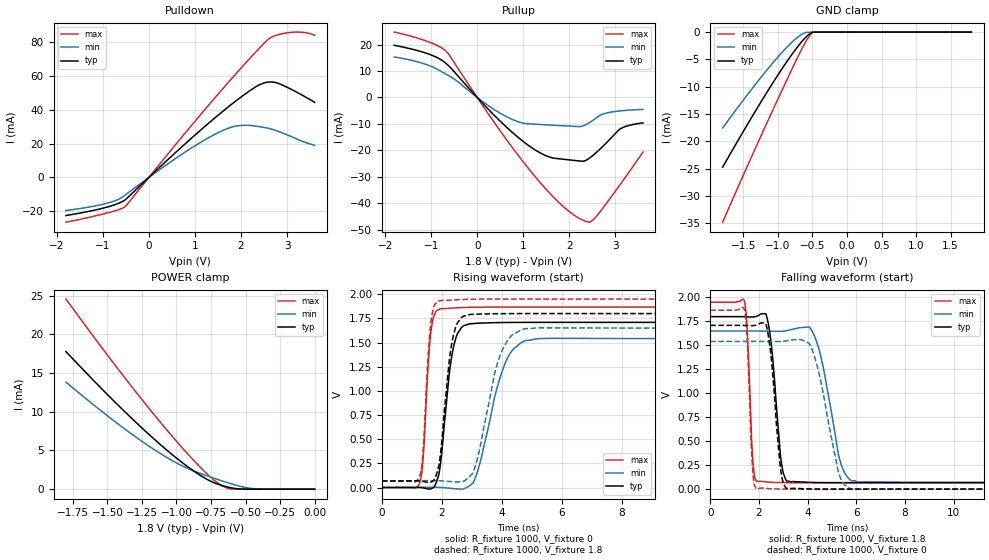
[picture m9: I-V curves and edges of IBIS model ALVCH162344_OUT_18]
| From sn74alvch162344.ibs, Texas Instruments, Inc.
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[Model]   ALVCH162344_OUT_18
Model_type  3-state
Enable   Active-Low
Vref =   0
Rref =   1000
Cref =   30p
Vmeas =   0.9
| variable   typ   min   max
C_comp   3.79pF   3.08pF   4.13pF
| C_pullup   2.49pF   1.20pF   4.61pF
| C_pulldown   1.14pF   0.73pF   1.99pF
| C_tri-state   3.79pF   3.08pF   4.13pF
[Temperature Range]   40   100   -40
| Ambient temperature   25   85   -40
[Voltage range]   1.8   1.65   1.95
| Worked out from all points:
|   slope of the pulldown table from 0 to 0.27 V, typ, clamps not added: 39.1 ohm
|   slope of the pullup table from 0 to 0.27 V, typ, clamps not added: 54.3 ohm
|   GND clamp passes 1 mA (typ) near -0.60 V on its own axis
|   POWER clamp passes 1 mA (typ) near -0.75 V on its own axis
|   rising waveform, R_fixture 1000, V_fixture 0: 20-80 % time 347ps typ, 732ps min, 205ps max; typ from 0 V to 1.71 V
|   falling waveform, R_fixture 1000, V_fixture 1.8: 20-80 % time 331ps typ, 662ps min, 179ps max; typ from 1.8 V to 0.067 V
|   rising waveform, R_fixture 1000, V_fixture 1.8: 20-80 % time 333ps typ, 654ps min, 202ps max; typ from 0.067 V to 1.8 V
|   falling waveform, R_fixture 1000, V_fixture 0: 20-80 % time 331ps typ, 716ps min, 170ps max; typ from 1.71 V to 0 V
[GND Clamp]
| ALVCH162344_OUT_18
|   Voltage   I(typ)   I(min)   I(max)
-1.8V     -24.75mA   -17.57mA   -34.84mA
-1.285V   -13.63mA   -8.929mA   -20.14mA
-1.08V    -9.446mA   -5.745mA   -14.47mA
-905mV    -6.056mA   -3.242mA   -9.706mA
-770mV    -3.623mA   -1.546mA   -6.073mA
-660mV    -1.839mA   -456.9uA   -3.236mA
-565mV    -568.6uA   -30.9uA    -1.109mA
-500mV    -40.16uA   -16.84uA   -114.6uA
-420mV    -2.964uA   -7.709uA   -1.366uA
1.8V      58.66pA    10.7nA     26.21pA
[POWER Clamp]
| ALVCH162344_OUT_18
|   Voltage   I(typ)   I(min)   I(max)
-1.8V     17.77mA    13.82mA    24.55mA
-1.44V    11.16mA    8.654mA    15.91mA
-1.15V    6.28mA     4.979mA    9.36mA
-1.015V   4.229mA    3.53mA     6.494mA
-900mV    2.655mA    2.525mA    4.186mA
-800mV    1.484mA    1.86mA     2.332mA
-715mV    735uA      1.33mA     985.6uA
-655mV    395.4uA    974.2uA    302.6uA
-605mV    178.9uA    695.8uA    24.81uA
-505mV    10.18uA    234.3uA    453nA
-425mV    558.3nA    44.67uA    18.74nA
-16.28fV  58.66pA    258.3pA    31.66pA
[Pulldown]
| ALVCH162344_OUT_18
|   Voltage   I(typ)   I(min)   I(max)
-1.8V     -22.48mA   -19.52mA   -26.42mA
-905mV    -17.49mA   -15.19mA   -20.95mA
-660mV    -15.29mA   -12.91mA   -19.09mA
-500mV    -12.91mA   -10.07mA   -16.79mA
660mV     16.68mA    12.65mA    22mA
1.47V     35.99mA    25.98mA    48.15mA
1.91V     45.59mA    30.44mA    61.8mA
2.415V    54.88mA    29.9mA     76.77mA
2.625V    56.36mA    28.8mA     82.2mA
2.885V    54.7mA     26.44mA    84.8mA
3.275V    49.39mA    21.93mA    85.78mA
3.6V      44.35mA    18.98mA    83.95mA
[Pullup]
| ALVCH162344_OUT_18
|   Voltage   I(typ)   I(min)   I(max)
-1.8V     19.73mA    15.31mA    24.72mA
-1.055V   16.43mA    12.16mA    21.02mA
-665mV    12.68mA    8.713mA    17.29mA
465mV     -8.372mA   -5.6mA     -11.78mA
1.115V    -18.15mA   -9.96mA    -26.89mA
1.59V     -22.62mA   -10.43mA   -36.47mA
2.27V     -24.1mA    -10.91mA   -46.19mA
2.44V     -22.89mA   -9.483mA   -47.15mA
2.565V    -21.14mA   -8.016mA   -45.39mA
2.755V    -18.03mA   -6.129mA   -41.21mA
3.105V    -11.9mA    -5.072mA   -32.9mA
3.6V      -9.595mA   -4.534mA   -20.62mA
[Ramp]
| ALVCH162344_OUT_18
| variable   typ   min   max
dV/dt_r   1.04/3.78E-10   0.94/7.80E-10   1.13/2.09E-10
dV/dt_f   1.06/3.45E-10   0.97/7.06E-10   1.15/1.95E-10
R_load = 1000
[Rising Waveform]
| ALVCH162344_OUT_18
R_fixture =   1000
C_fixture =   0
L_fixture =   0
V_fixture =   0
V_fixture_min = 0
V_fixture_max = 0
|   Time   V(typ)   V(min)   V(max)
0s        23.14uV    37.1uV     16.41uV
1.265ns   1.49mV     443.1uV    50.96mV
1.38ns    -3.025mV   1.424mV    312.9mV
1.635ns   -13.16mV   2.091mV    1.605V
1.955ns   243.9mV    885.8uV    1.85V
2.375ns   1.429V     -10.55mV   1.857V
2.915ns   1.693V     15.15mV    1.865V
4.115ns   1.708V     1.288V     1.867V
4.83ns    1.709V     1.522V     1.867V
24.99ns   1.709V     1.541V     1.867V
[Falling Waveform]
| ALVCH162344_OUT_18
R_fixture =   1000
C_fixture =   0
L_fixture =   0
V_fixture =   1.8
V_fixture_min = 1.65
V_fixture_max = 1.95
|   Time   V(typ)   V(min)   V(max)
0s        1.8V       1.65V      1.95V
1.405ns   1.799V     1.65V      1.963V
1.745ns   1.796V     1.65V      332.3mV
1.915ns   1.804V     1.65V      78.89mV
2.395ns   1.716V     1.648V     73.8mV
2.895ns   336.1mV    1.646V     68.42mV
3.17ns    81.25mV    1.655V     67.67mV
4.28ns    69.18mV    1.601V     67.01mV
5.82ns    67.3mV     87.47mV    67.19mV
24.99ns   67.42mV    70.3mV     67.21mV
[Rising Waveform]
| ALVCH162344_OUT_18
R_fixture =   1000
C_fixture =   0
L_fixture =   0
V_fixture =   1.8
V_fixture_min = 1.65
V_fixture_max = 1.95
|   Time   V(typ)   V(min)   V(max)
0s        67.38mV    70.2mV     67.19mV
1.265ns   68.15mV    70.35mV    121.6mV
1.375ns   63.91mV    71.16mV    377.1mV
1.62ns    54.23mV    71.39mV    1.667V
1.885ns   205.2mV    70.09mV    1.932V
2.355ns   1.528V     60.34mV    1.941V
2.905ns   1.789V     105.3mV    1.948V
3.95ns    1.799V     1.37V      1.95V
4.755ns   1.8V       1.641V     1.95V
24.99ns   1.8V       1.65V      1.95V
[Falling Waveform]
| ALVCH162344_OUT_18
R_fixture =   1000
C_fixture =   0
L_fixture =   0
V_fixture =   0
V_fixture_min = 0
V_fixture_max = 0
|   Time   V(typ)   V(min)   V(max)
0s        1.709V     1.541V     1.867V
1.4ns     1.708V     1.541V     1.879V
1.735ns   1.706V     1.541V     238.5mV
1.905ns   1.713V     1.541V     579uV
2.365ns   1.638V     1.541V     6.197mV
2.88ns    228.7mV    1.541V     997.2uV
3.145ns   6.755mV    1.548V     356.6uV
4.16ns    1.561mV    1.472V     -205.1uV
5.765ns   -147.9uV   4.211mV    -18.49uV
24.99ns   237.8nV    402.4nV    184.9nV
